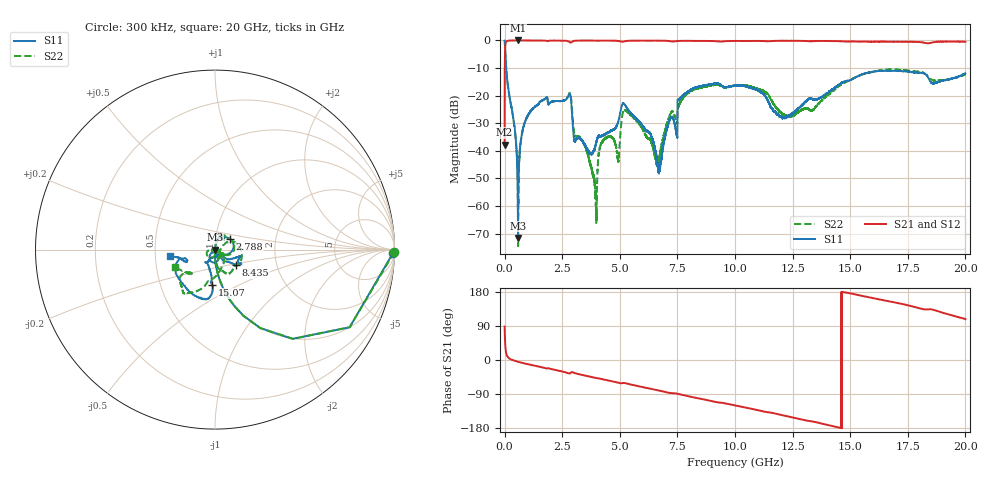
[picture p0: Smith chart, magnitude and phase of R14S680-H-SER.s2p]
!{R14S680}
!Johanson Technology Inc.
!www.johansontechnology.com
!Test Board Conditions:
!Substrate Type  RO4350B
!Substrate Thickness  20 mil
!Substrate Dk  3.66
!TL Type: GCPW
!TL Trace Width  36 mil
!TL Gap  12 mil
!Electrode orientation  Horizontal
!DUT TOPOLOGY	SERIES
!Mounting Pad LxW  26x36 mil
! Created Wed Nov 25 17:33:21 2020
! 2 Port Network Data from SP1.SP block
! freq  magS11  angS11  magS21  angS21  magS12  angS12  magS22  angS22
# khz S ma R 50
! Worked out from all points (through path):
!   20001 points, 300 kHz to 20 GHz, reference 50 ohm
!   highest |S21| = 0.00 dB at 579.3 MHz (marker M1); lowest = -37.7 dB at 300 kHz (marker M2)
!   group delay of S21, straight-line fit = 34.8 ps
!   lowest |S11| = -71.5 dB at 583.3 MHz (marker M3), VSWR 1.00, Z = 50 - j0.00716 ohm
!   |S11| at or under -10 dB: 68.48 MHz to end of sweep
!   |S22| runs from -74.5 to 0.0 dB; largest |S21 - S12| = 0.018
!   S11 on the Smith chart (normalised r, x): 300 kHz: open; 2.788 GHz: 1.17, +0.14; 8.435 GHz: 1.25, -0.22; 15.07 GHz: 0.90, -0.37; 20 GHz: 0.60, -0.05
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300  0.9933 -1.0  0.01303 88.3  0.01298 89.2  0.998 -0.9
112300  0.1952 -79.6  0.9803 10.3  0.9797 10.2  0.1962 -79.7
579300  0.0007826 -113.5  1 -4.7  0.9989 -4.6  0.001024 -92.7
583300  0.0002647 -164.3  0.9999 -4.8  0.9991 -4.8  0.0006127 -73.8
1116300  0.05151 78.3  0.9973 -12.5  0.9977 -12.5  0.05115 75.9
2788300  0.1016 36.2  0.9584 -35.5  0.958 -35.5  0.1049 31.9
3052300  0.01498 17.6  0.9864 -34.5  0.9865 -34.6  0.01906 3.4
3334300  0.01598 40.1  0.9949 -39.0  0.9958 -39.0  0.01604 36.0
3930300  0.01183 -41.0  0.9931 -47.0  0.9927 -47.0  0.002042 100.7
4193300  0.01871 -88.3  0.9933 -49.9  0.9931 -49.9  0.01369 -165.5
4912300  0.03192 -70.1  0.9827 -59.9  0.9821 -59.9  0.006951 -155.3
5186300  0.07097 -104.6  0.9608 -60.8  0.9603 -60.8  0.0542 -130.5
6328300  0.02049 -135.3  0.9892 -75.6  0.9905 -75.7  0.01569 -155.0
6667300  0.004878 -102.1  0.9926 -80.2  0.9919 -80.2  0.006296 -75.0
7600300  0.08786 -47.5  0.9812 -90.4  0.9811 -90.4  0.07155 31.5
8435300  0.1454 -35.8  0.9788 -101.4  0.9788 -101.4  0.1349 7.5
1.00003e7  0.1524 -14.4  0.9786 -119.8  0.9788 -119.8  0.1509 -50.1
1.21123e7  0.04073 -73.9  0.9865 -146.4  0.9886 -146.4  0.04553 -54.1
1.33343e7  0.08781 -127.8  0.9684 -162.1  0.9698 -162.1  0.05333 -42.5
1.50703e7  0.1973 -94.3  0.9596 175.1  0.9626 174.9  0.1977 -104.3
1.66673e7  0.279 -105.7  0.9511 155.1  0.9423 154.9  0.2977 -124.8
2e7  0.2528 -171.2  0.9474 108.1  0.9467 108.2  0.2439 -157.0
